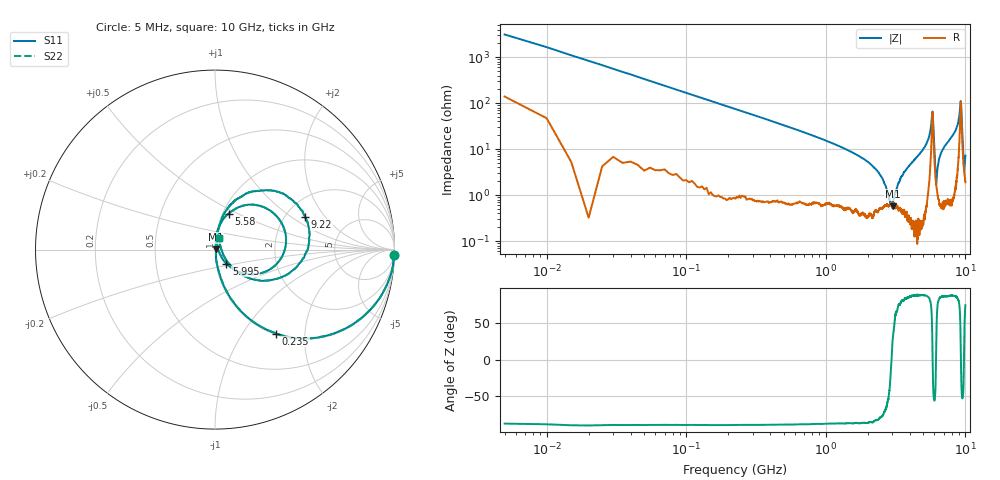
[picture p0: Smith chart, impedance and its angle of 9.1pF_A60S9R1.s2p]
! Amotech Co.,Ltd.
! http://www.amotech.co.kr/
! Part Number: A60S9R1
! These Parameters are Measured in Series Mode Connection
! Operation Temp=25[degC], DC Bias Voltage=0[V]
! Freq. Start=5[MHz] Stop=10[GHz], 2000[Steps]
! Date: Monday, July 13, 2020, 01:34:07
# GHZ S RI R 50.000000
!Freq.(Hz) S11(Real) S11(Imag) S21(Real) S21(Imag) S12(Real) S12(Imag) S22(Real) S22(Imag)
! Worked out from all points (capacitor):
!   2000 points, 5 MHz to 10 GHz, reference 50 ohm
!   read as one part in series: C = 9.46 pF near 55 MHz
!   lowest |Z| = 570 mohm at 3.005 GHz (marker M1)
!   series resonance near 2.956 GHz, so ESL is about 310 pH
!   S11 on the Smith chart (normalised r, x): 5 MHz: 4, -63; 235 MHz: 1.02, -1.43; 5.58 GHz: 1.07, +0.45; 5.995 GHz: 1.12, -0.18; 9.22 GHz: 2.55, +1.30; 10 GHz: 1.04, +0.14
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0.005  0.9976 -0.0318  0.00244 0.0318  0.00244 0.0318  0.9976 -0.0318
0.09  0.7745 -0.4115  0.2255 0.4115  0.2255 0.4115  0.7745 -0.4115
0.235  0.3412 -0.468  0.6588 0.468  0.6588 0.468  0.3412 -0.468
0.59  0.0772 -0.2555  0.9228 0.2555  0.9228 0.2555  0.0772 -0.2555
1.675  0.0101 -0.0735  0.9899 0.0735  0.9899 0.0735  0.0101 -0.0735
2.395  0.00557 -0.0299  0.9944 0.0299  0.9944 0.0299  0.00557 -0.0299
3.005  0.00514 0.00238  0.9949 -0.00238  0.9949 -0.00238  0.00514 0.00238
3.34  0.00534 0.0183  0.9947 -0.0183  0.9947 -0.0183  0.00534 0.0183
5.005  0.0126 0.1003  0.9874 -0.1003  0.9874 -0.1003  0.0126 0.1003
5.58  0.0758 0.2006  0.9242 -0.2006  0.9242 -0.2006  0.0758 0.2006
5.725  0.2279 0.2483  0.7721 -0.2483  0.7721 -0.2483  0.2279 0.2483
5.815  0.3954 0.0357  0.6046 -0.0357  0.6046 -0.0357  0.3954 0.0357
5.995  0.0628 -0.078  0.9372 0.078  0.9372 0.078  0.0628 -0.078
6.18  0.0164 0.00492  0.9836 -0.00492  0.9836 -0.00492  0.0164 0.00492
6.38  0.0105 0.045  0.9895 -0.045  0.9895 -0.045  0.0105 0.045
6.67  0.0122 0.0785  0.9878 -0.0785  0.9878 -0.0785  0.0122 0.0785
8.335  0.0578 0.2125  0.9422 -0.2125  0.9422 -0.2125  0.0578 0.2125
8.895  0.1623 0.3043  0.8377 -0.3043  0.8377 -0.3043  0.1623 0.3043
9.22  0.5026 0.1816  0.4974 -0.1816  0.4974 -0.1816  0.5026 0.1816
9.405  0.2961 -0.172  0.7039 0.172  0.7039 0.172  0.2961 -0.172
9.775  0.0347 0.00367  0.9653 -0.00367  0.9653 -0.00367  0.0347 0.00367
10  0.0232 0.0665  0.9768 -0.0665  0.9768 -0.0665  0.0232 0.0665
